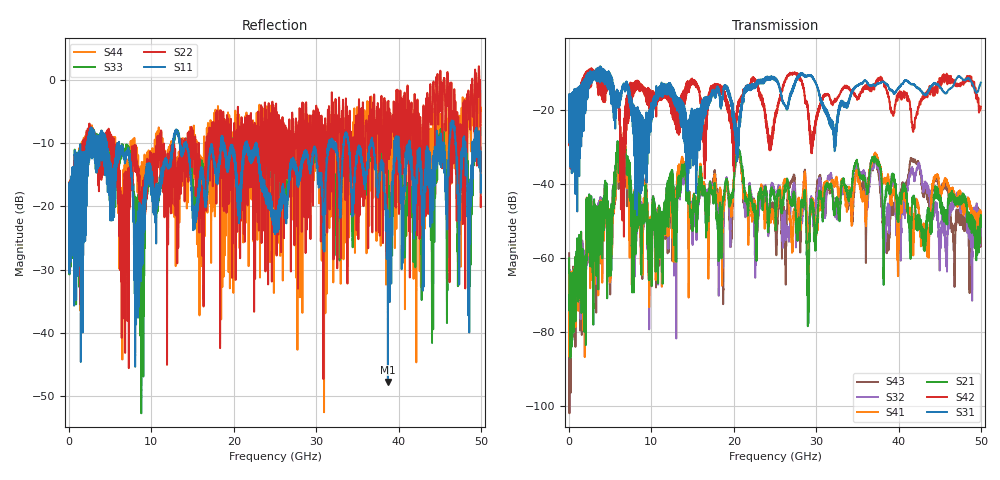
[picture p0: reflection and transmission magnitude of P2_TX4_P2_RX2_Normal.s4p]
!Keysight Technologies,N5225B,MY57041031,A.13.20.10
!Date: Friday, May 31, 2019 11:29:19
!Correction: S11(Full 4 Port(1,2,3,4))
!S12(Full 4 Port(1,2,3,4))
!S13(Full 4 Port(1,2,3,4))
!S14(Full 4 Port(1,2,3,4))
!S21(Full 4 Port(1,2,3,4))
!S22(Full 4 Port(1,2,3,4))
!S23(Full 4 Port(1,2,3,4))
!S24(Full 4 Port(1,2,3,4))
!S31(Full 4 Port(1,2,3,4))
!S32(Full 4 Port(1,2,3,4))
!S33(Full 4 Port(1,2,3,4))
!S34(Full 4 Port(1,2,3,4))
!S41(Full 4 Port(1,2,3,4))
!S42(Full 4 Port(1,2,3,4))
!S43(Full 4 Port(1,2,3,4))
!S44(Full 4 Port(1,2,3,4))
!S4P File: Measurements: <S11,S12,S13,S14>,
!<S21,S22,S23,S24>,
!<S31,S32,S33,S34>,
!<S41,S42,S43,S44>:
# Hz S  dB  R 50.0
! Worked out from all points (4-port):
!   5000 points, 10 MHz to 50 GHz, reference 50 ohm
!   strongest paths, dB at 10 MHz, 12.51 GHz, 25.01 GHz, 37.51 GHz, 50 GHz:
!     S31: -19.3, -14.3, -11.3, -12.8, -12.5
!     S42: -19.5, -15.9, -22.0, -11.8, -19.1
!     S21: -60.1, -41.8, -46.4, -34.4, -49.8
!     S41: -62.2, -42.0, -50.4, -33.1, -49.7
!     S32: -62.5, -43.4, -43.8, -35.4, -53.8
!     S43: -58.7, -43.1, -50.5, -36.0, -54.0
!   lowest |S11| = -47.8 dB at 38.71 GHz (marker M1), VSWR 1.01, Z = 49.6 + j0.0116 ohm
!   |S11| at or under -10 dB: 6.073 GHz to 12.61 GHz (6.542 GHz wide, 70 % of centre); 14.21 GHz to 18.43 GHz (4.227 GHz wide, 25.9 % of centre); 22.71 GHz to 31.52 GHz (8.805 GHz wide, 32.5 % of centre)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
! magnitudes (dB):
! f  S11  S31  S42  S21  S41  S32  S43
! 10 MHz  -19.0  -19.3  -19.5  -60.1  -62.2  -62.5  -58.7
! 6.63 GHz  -12.4  -13.5  -26.1  -28.7  -28.6  -29.2  -29.2
! 9.78 GHz  -13.2  -22.3  -14.8  -65.2  -61.7  -63.4  -61.3
! 20.52 GHz  -21.0  -27.9  -18.2  -31.3  -31.4  -31.9  -31.9
! 29.01 GHz  -11.9  -10.7  -19.7  -65.7  -61.7  -52.9  -55.6
! 38.71 GHz  -47.8  -13.5  -15.3  -40.0  -37.4  -45.2  -54.4
! 50 GHz  -15.0  -12.5  -19.1  -49.8  -49.7  -53.8  -54.0
